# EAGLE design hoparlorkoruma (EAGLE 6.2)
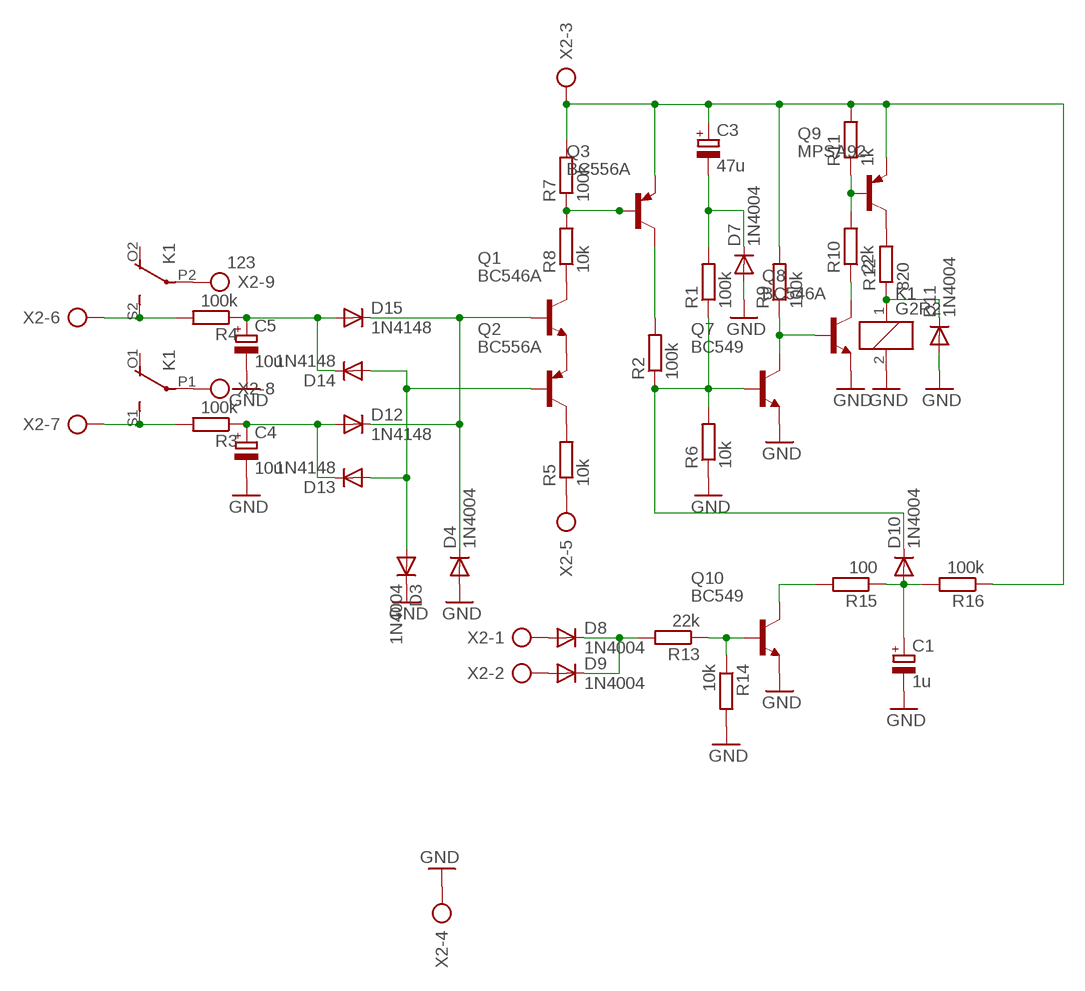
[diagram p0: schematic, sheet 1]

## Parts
C1  1u  CPOL-EUE2.5-6  [E2,5-6]
C3  47u  CPOL-EUE5-8.5  [E5-8,5]
C4  10u  CPOL-EUE2.5-6  [E2,5-6]
C5  10u  CPOL-EUE2.5-6  [E2,5-6]
D3  1N4004  [DO41-10]
D4  1N4004  [DO41-10]
D7  1N4004  [DO41-10]
D8  1N4004  [DO41-10]
D9  1N4004  [DO41-10]
D10  1N4004  [DO41-10]
D11  1N4004  [DO41-10]
D12  1N4148  1N4148DO35-10  [DO35-10]
D13  1N4148  1N4148DO35-7  [DO35-7]
D14  1N4148  1N4148DO35-10  [DO35-10]
D15  1N4148  1N4148DO35-10  [DO35-10]
K1  G2R2  [G2R2]
Q1  BC546A  [TO92-EBC]
Q2  BC556A  [TO92-EBC]
Q3  BC556A  [TO92-EBC]
Q7  BC549  BC546A  [TO92-EBC]
Q8  BC546A  [TO92-EBC]
Q9  MPSA92  MPSA56  [TO92-CBE]
Q10  BC549  BC546A  [TO92-EBC]
R1  100k  R-EU_0207/10  [0207/10]
R2  100k  R-EU_0207/10  [0207/10]
R3  100k  R-EU_0207/10  [0207/10]
R4  100k  R-EU_0207/10  [0207/10]
R5  10k  R-EU_0207/10  [0207/10]
R6  10k  R-EU_0207/10  [0207/10]
R7  100k  R-EU_0207/10  [0207/10]
R8  10k  R-EU_0207/10  [0207/10]
R9  100k  R-EU_0207/10  [0207/10]
R10  22k  R-EU_0207/10  [0207/10]
R11  1k  R-EU_0207/10  [0207/10]
R12  820  R-EU_0411/15  [0411/15]
R13  22k  R-EU_0207/10  [0207/10]
R14  10k  R-EU_0207/10  [0207/10]
R15  100  R-EU_0207/10  [0207/10]
R16  100k  R-EU_0207/10  [0207/10]
X2  123  AK500/9  [AK500/9]

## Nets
GND: C1.- C4.- C5.- D3.C D4.A D7.A D11.A K1.2 Q7.E Q8.E Q10.E R6.1 R14.2 X2.4
N$1: Q1.E Q2.E
N$2: Q2.C R5.2
N$3: Q1.C R8.1
N$4: Q3.B R7.1 R8.2
N$5: C5.+ D14.C D15.A R4.1
N$6: C4.+ D12.A D13.C R3.1
N$7: D4.C D12.C D15.C Q1.B
N$8: D3.A D13.A D14.A Q2.B
N$9: Q7.C Q8.B R9.1
N$10: Q9.B R10.2 R11.1
N$11: C3.+ Q3.E Q9.E R7.2 R9.2 R11.2 R16.1 X2.3
N$12: Q3.C R2.2
N$13: D10.C Q7.B R1.1 R2.1 R6.2
N$14: C3.- D7.C R1.2
N$15: Q9.C R12.2
N$16: Q8.C R10.1
N$17: Q10.B R13.1 R14.1
N$18: D8.C D9.C R13.2
N$19: D8.A X2.1
N$20: Q10.C R15.2
N$21: C1.+ D10.A R15.1 R16.2
N$22: D9.A X2.2
N$23: R5.1 X2.5
N$24: K1.S2(3:S) R4.2 X2.6
N$25: K1.S1(2:S) R3.2 X2.7
N$26: K1.P2(3:P) X2.9
N$27: K1.P1(2:P) X2.8
N$28: D11.C K1.1 R12.1
Unconnected: K1.O1(2:O) K1.O2(3:O)

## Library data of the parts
C1 C3-C5 = rcl:CPOL-EU: POLARIZED CAPACITOR, European symbol
D3 D4 D7-D11 = diode:1N4004: DIODE
D12-D15 = diode:1N4148: DIODE
K1 = relay:G2R2: RELAY 2 x switch, Omron; MF: OMRON COMPONENTS USA; MPN: G2R-2-DC6; OC_FARNELL: unknown; OC_NEWARK: 89C5317
Q1 Q7 Q8 Q10 = transistor-npn:BC546*: NPN Transistor
Q2 Q3 = transistor-pnp:BC556*: PNP Transistror
Q9 = transistor-pnp:MPSA56*: PNP Transistror Source: http://www.fairchildsemi.com/ds/MM/MMBTA56.pdf
R1-R16 = LME49810:R-EU_: RESISTOR, European symbol
X2 = con-ptr500:AK500/9: CONNECTOR; OC_FARNELL: unknown; OC_NEWARK: unknown

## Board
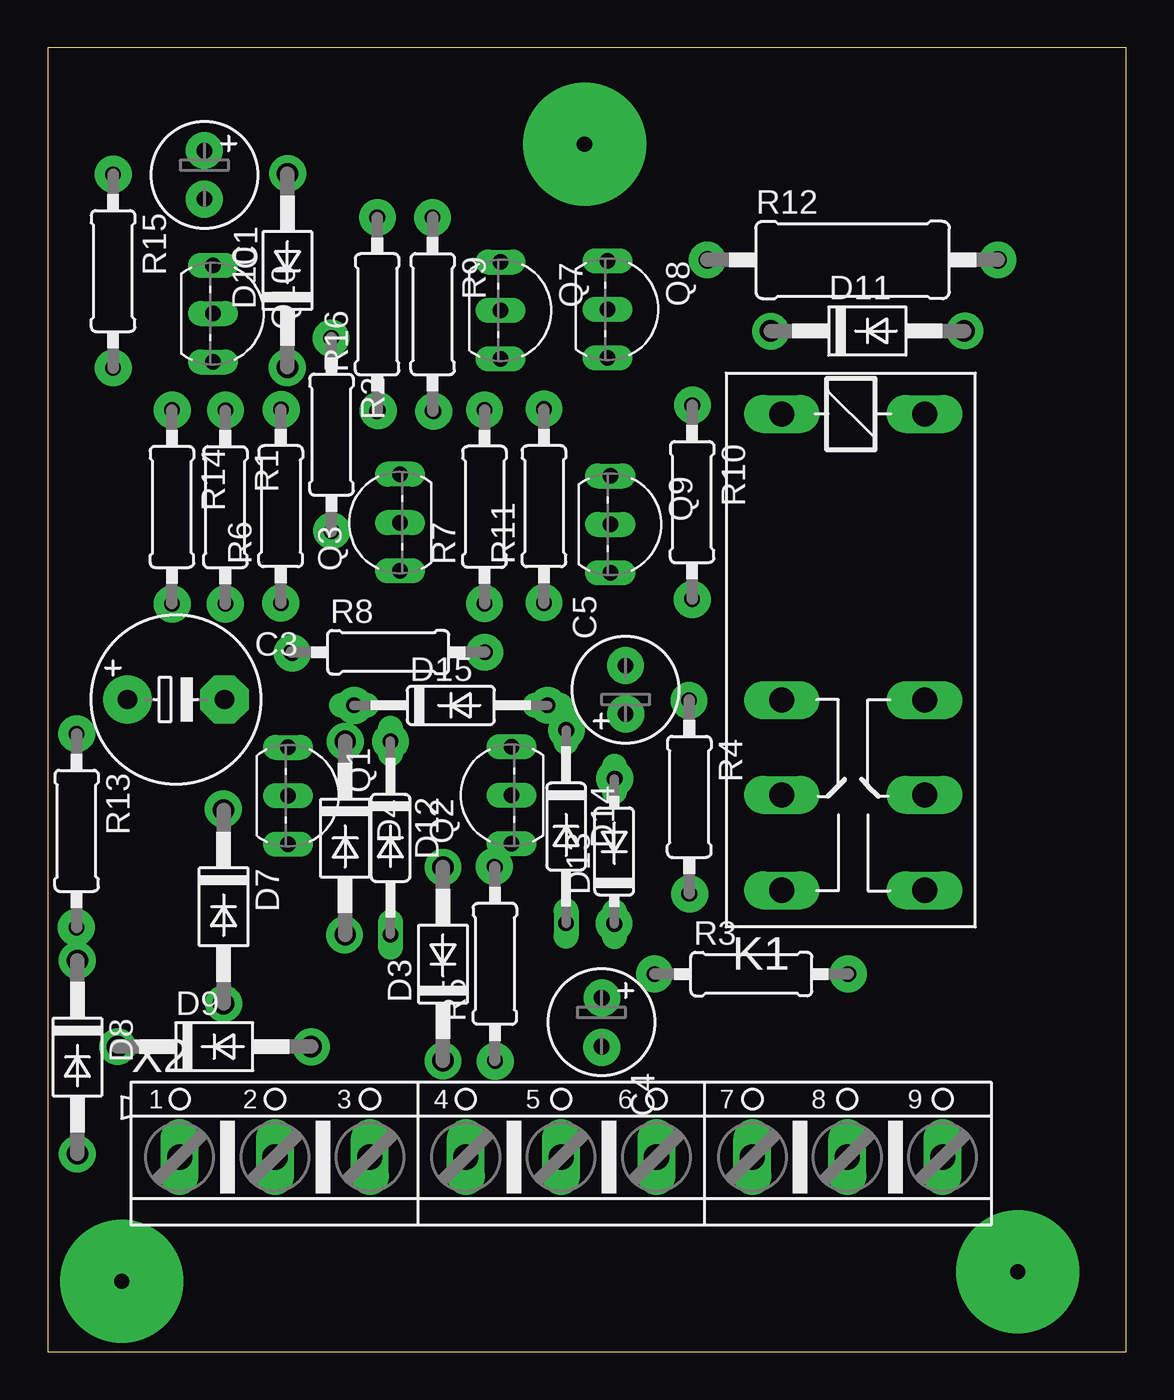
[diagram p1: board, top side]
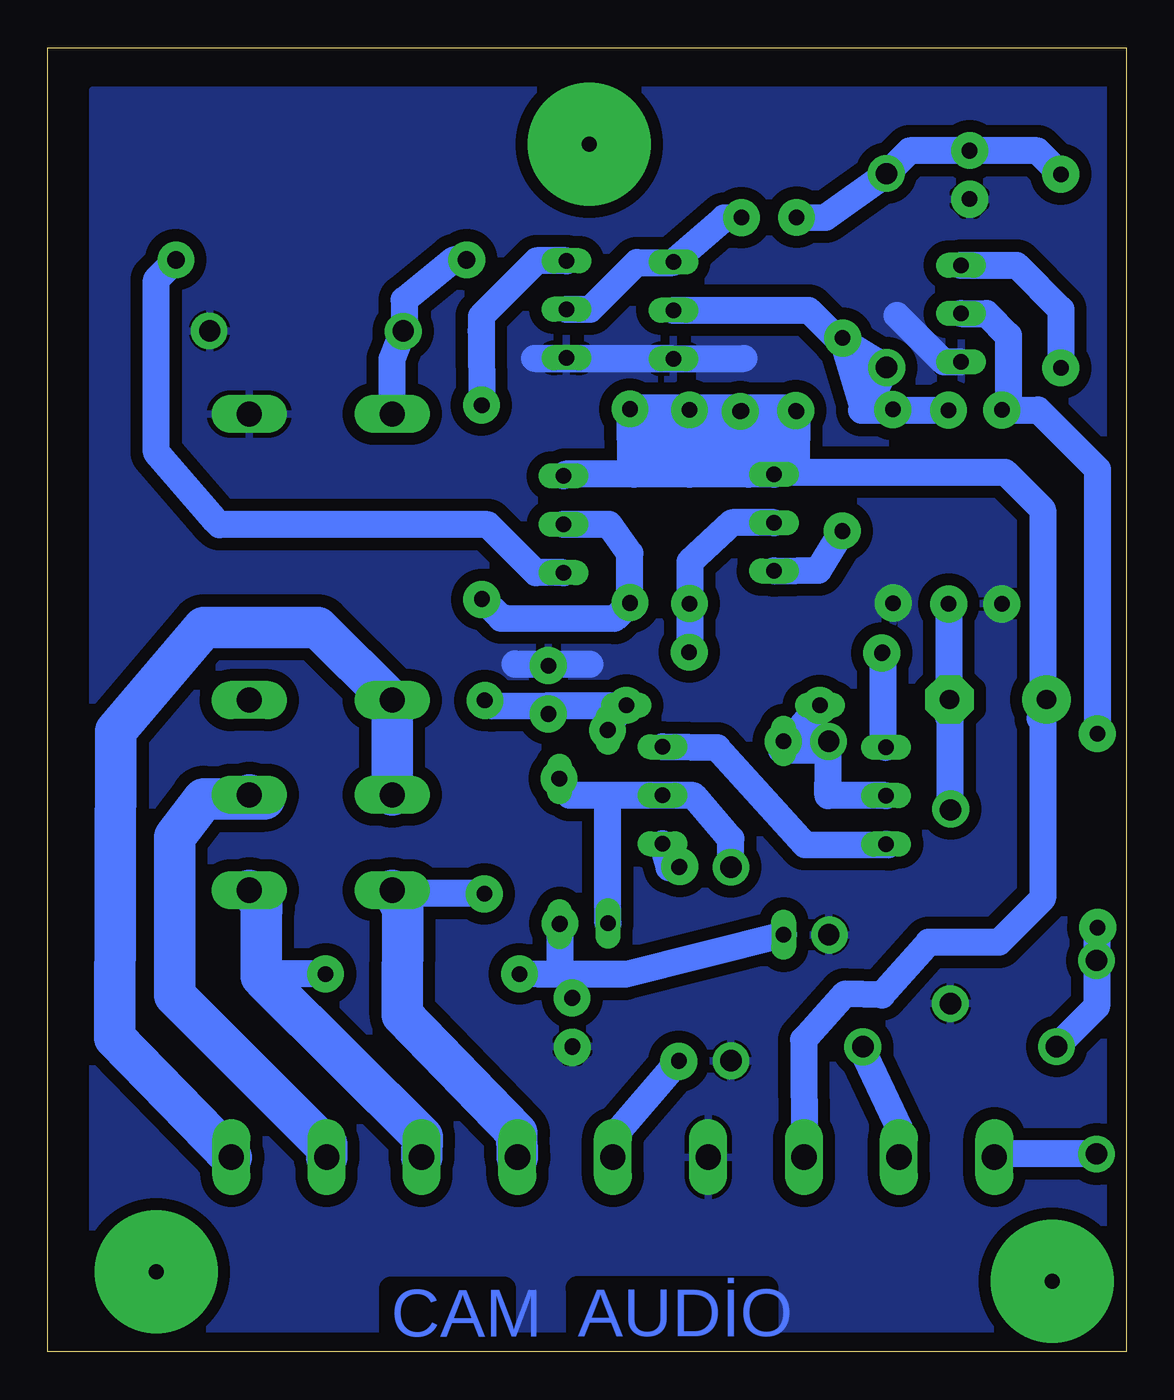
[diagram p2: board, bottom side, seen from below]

Size 56.59 x 68.45 mm. Coordinates in mm from the lower left corner, seen from the top.
Outline: 0,0 56.59,0 56.59,68.45 0,68.45 0,0
Copper layers (1*16): Top 0.035mm / dielectric 1.5mm / Bottom 0.035mm
Design rules: minimum track width 10mil, minimum drill 24mil, track to track 25mil, track to pad 25mil, pad to pad 25mil, via to via 25mil, smd to smd 25mil, copper to edge 40mil, drill to drill 8mil, minimum pad ring 10mil, minimum via ring 8mil, stop-mask expansion 4mil, vias tented up to drill 0mil, thermal gap 10mil

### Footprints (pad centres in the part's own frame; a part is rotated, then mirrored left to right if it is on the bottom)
E2,5-6 = drill 0.813 pad 1.6: + -1.27,0 | drill 0.813 pad 1.6 octagon: - 1.27,0
E5-8,5 = drill 1.016 pad 2.54: + -2.54,0 | drill 1.016 pad 2.54 octagon: - 2.54,0
DO41-10 = drill 1.118: A 5.08,0; C -5.08,0
DO35-10 = drill 0.813 long: A 5.08,0; C -5.08,0
DO35-7 = drill 0.813 long: A 3.81,0; C -3.81,0
G2R2 = drill 1.321 long: 1 -2.54,-3.683; 2 -2.54,3.81; O1 12.471,3.81; O2 12.471,-3.683; P1 17.45,3.81; P2 17.45,-3.683; S1 22.454,3.81; S2 22.454,-3.683
TO92-EBC = drill 0.813 long: B 0,-1.27; C -2.54,-1.27; E 2.54,-1.27
TO92-CBE = drill 0.813 long: B 0,0; C 2.54,0; E -2.54,0
0207/10 = drill 0.813 octagon: 1 -5.08,0; 2 5.08,0
0411/15 = drill 0.914 octagon: 1 -7.62,0; 2 7.62,0
AK500/9 = drill 1.321 long: 1 -20.015,0; 2 -15.011,0; 3 -10.033,0; 4 -5.004,0; 5 0,0; 6 5.004,0; 7 10.033,0; 8 15.011,0; 9 20.015,0

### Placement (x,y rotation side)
C1  8.22,61.77 270 top
C3  6.73,34.24 0 top
C4  29.05,17.31 270 top
C5  30.32,34.75 90 top
D3  20.74,20.36 90 top
D4  15.61,26.97 270 top
D7  9.23,23.36 270 top
D8  1.56,15.47 270 top
D9  8.74,16.02 0 top
D10  12.58,56.75 90 top
D11  43.01,53.58 0 top
D12  17.98,26.98 270 top
D13  29.73,26.26 90 top
D14  27.2,27.57 270 top
D15  21.15,33.93 0 top
K1  42.2,46.68 270 top
Q1  13.88,29.19 270 top
Q2  23.07,29.21 90 top
Q3  17.21,43.52 90 top
Q7  25.03,54.66 270 top
Q8  30.64,54.72 270 top
Q9  29.52,43.43 270 top
Q10  9.94,54.49 270 top
R1  9.32,44.33 270 top
R2  14.89,48.14 270 top
R3  36.92,19.83 0 top
R4  33.66,29.13 270 top
R5  23.46,20.37 90 top
R6  12.23,44.38 90 top
R7  22.92,44.35 90 top
R8  17.86,36.72 0 top
R9  20.2,54.46 270 top
R10  33.81,44.6 270 top
R11  26.04,44.38 90 top
R12  42.23,57.31 0 top
R13  1.52,27.35 270 top
R14  6.52,44.35 270 top
R15  3.43,56.72 270 top
R16  17.29,54.45 90 top
X2  26.94,10.22 0 top

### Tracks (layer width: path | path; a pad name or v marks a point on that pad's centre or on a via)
GND  (via drill 0.8 pad 1.93)
  Bottom 1.422: v6.53,39.25 R14.2 | 12.19,39.26 R6.1 | C4.- v29.07,15.98 | Q7.E 31.04,52.14 20.05,52.14 | 28.13,36.09 32.07,36.09 32.07,36.11 | 8.69,51.95 9.57,51.95 12.03,54.41
  other vias: 12.23,39.3 15.57,21.89 20.74,15.28 30.32,36.02 9.24,18.28 48.13,53.58 8.22,60.49
  pour Bottom: 0.7,66.22 54.23,66.22 54.23,0.51 0.7,0.51
N$1
  Bottom 1.422: Q1.E 12.47,26.61 16.86,26.62 21.45,31.7 Q2.E
N$2
  Bottom 1.422: Q2.C 23.98,25.4 R5.2
N$3
  Bottom 1.422: R8.1 12.78,31.9 arc-90 Q1.C
N$4  (via drill 0.8 pad 1.93)
  Bottom 1.422: Q3.B 20.68,43.52 22.89,41.46 22.89,39.25 | 22.89,39.25 22.89,36.77 R8.2 | R7.1 22.89,39.25
  other vias: 22.92,39.27
N$5
  Bottom 1.422: 27.32,32.77 D14.C 27.2,32.96 D15.A 30.36,33.91 | R4.1 33.28,33.9 30.36,33.91 | C5.+ 30.32,33.87 30.36,33.91
N$6
  Bottom 1.422: D12.A 26.3,19.82 28.37,19.81 | 28.37,19.81 30.82,19.82 31.93,19.84 | 31.93,19.84 R3.1 | D13.C 29.73,19.82 31.93,19.84 | C4.+ 29.05,19.77 28.37,19.81
N$7
  Bottom 1.422: Q1.B 15.66,29.19 D4.C 17.62,32.48 15.77,31.57 | D12.C 15.77,31.57 | D15.C 18.1,31.58 15.77,31.57
N$8
  Bottom 1.422: D3.A 20.74,26.93 22.7,29.2 Q2.B 27.06,29.21 | 27.06,29.21 29.2,29.21 D13.A | D14.A 27.2,29.07 27.06,29.21
N$9
  Bottom 1.422: R9.1 21.1,59.51 Q7.C 23.79,57.17 25.68,57.17 28.13,54.72 Q8.B
N$10
  Bottom 1.422: Q9.B 27.13,43.42 26.04,41.91 R11.1 26.84,38.49 32.55,38.51 32.8,38.51 R10.2
N$11
  Bottom 1.422: 17.39,46.17 18.37,46.17 Q3.E 19.83,46.06 | 17.39,46.17 6.36,46.17 4.39,44.2 4.39,33.12 | 16.89,10.22 X2.3 16.93,16.38 14.77,18.78 12.82,18.73 10.37,21.5 6.69,21.5 4.39,23.8 4.39,33.12 | C3.+ 4.52,33.25 4.39,33.12 | 19.83,46.06 22.91,46.06 | 22.91,46.06 25.82,46.06 | 25.82,46.06 29.43,46.06 Q9.E | R11.2 26.02,46.21 25.82,46.06 | R7.2 22.84,46.13 22.91,46.06 | R9.2 19.91,46.14 19.83,46.06 | R16.1 17.32,46.24 17.39,46.17
N$12
  Bottom 1.422: Q3.C 16.14,41.02 R2.2
N$13  (via drill 0.8 pad 1.93)
  Bottom 1.422: R1.1 12.39,49.41 | 12.39,49.41 13.89,49.41 | 13.89,49.41 13.83,49.63 R2.1 | R6.2 v12.25,49.46 12.34,49.46 12.39,49.41 | 13.89,49.41 13.62,49.68 D10.C 13.07,51.97 | 15.1,53.23 13.07,51.97 | Q7.B 16.66,54.66 13.38,51.38 13.38,51.66 13.07,51.97
N$14
  Bottom 1.422: R1.2 9.32,33.31 C3.- 9.23,34.2 D7.C
N$15
  Bottom 1.422: 47.77,43.58 47.88,43.71 | 47.88,43.71 50.89,47.2 50.89,56.27 R12.2 | 47.88,43.71 47.58,43.41 33.5,43.41 30.98,40.89 Q9.C
N$16
  Bottom 1.422: R10.1 33.85,53.58 33.84,53.59 33.84,54.35 30.93,57.26 Q8.C
N$17
  Bottom 1.422: 6.39,49.56 R14.1 | R14.1 4.62,49.43 1.52,46.33 R13.1 | Q10.B 7.33,54.49 6.18,53.34 6.18,49.77 R14.1
N$18
  Bottom 1.422: D9.C 1.56,18.12 D8.C 1.56,22.23 R13.2
N$19
  Bottom 1.422: D8.A 6.75,10.39 X2.1
N$20
  Bottom 1.422: Q10.C 5.76,57.03 3.43,54.7 R15.2
N$21
  Bottom 1.422: 12.85,61.75 D10.A | R16.2 15.78,59.54 D10.A | R15.1 4.67,63.04 C1.+ 11.37,63.04 D10.A
N$22
  Bottom 1.422: 11.93,10.34 X2.2 11.89,10.26 11.89,11.7 13.66,15.47 D9.A
N$23
  Bottom 1.422: R5.1 26.94,11.23 X2.5
N$24
  Bottom 1.422: R4.2 37.93,24.05 38.23,23.74
  Bottom 2.184: X2.6 31.97,11.49 37.98,17.68 37.95,23.26 38.23,23.74 K1.S2
N$25
  Bottom 1.422: 45.37,23.13 45.39,23.11 | R3.2 44.69,19.83 45.12,19.41
  Bottom 2.184: X2.7 36.94,11.29 45.12,19.41 45.39,19.7 45.39,23.11 | K1.S1 45.37,23.59 45.37,23.13
N$26
  Bottom 2.184: K1.P2 38.52,34.13 42.41,38.02 48.41,38.02 53.03,32.58 53.06,16.48 X2.9
N$27
  Bottom 2.184: X2.8 41.95,10.74 | 41.95,10.74 41.95,10.88 | K1.P1 45.22,29.02 48.41,29.02 49.91,27.02 49.91,18.7 41.95,10.74
N$28  (via drill 0.8 pad 1.93)
  Bottom 1.422: K1.1 38.52,52.1 D11.C 37.89,53.62 37.89,55.2 35.28,57.31 R12.1
  other vias: 34.61,57.31
N$29  (via drill 0.8 pad 6.45)
  other vias: 3.89,3.7
N$30  (via drill 0.8 pad 6.45)
  other vias: 50.89,4.2
N$31  (via drill 0.8 pad 6.45)
  other vias: 28.17,63.38
N$32  (via drill 0.8 pad 1.93)
  other vias: 1.5,22.27
N$33  (via drill 0.8 pad 1.93)
  other vias: 1.52,32.44
N$34  (via drill 0.8 pad 1.93)
  other vias: 6.54,49.43
N$35  (via drill 0.8 pad 1.93)
  other vias: 9.33,49.43
N$36  (via drill 0.8 pad 1.93)
  other vias: 14.87,53.21
N$37  (via drill 0.8 pad 1.93)
  other vias: 17.34,49.4
N$38  (via drill 0.8 pad 1.93)
  other vias: 20.26,49.36
N$39  (via drill 0.8 pad 1.93)
  other vias: 12.57,51.66
N$40  (via drill 0.8 pad 1.93)
  other vias: 3.44,51.64
N$41  (via drill 0.8 pad 1.93)
  other vias: 3.44,61.81
N$42  (via drill 0.8 pad 1.93)
  other vias: 12.6,61.85
N$43  (via drill 0.8 pad 1.93)
  other vias: 17.3,59.54
N$44  (via drill 0.8 pad 1.93)
  other vias: 20.19,59.53
N$45  (via drill 0.8 pad 1.93)
  other vias: 33.83,49.69
N$46  (via drill 0.8 pad 1.93)
  other vias: 26.04,49.49
N$47  (via drill 0.8 pad 1.93)
  other vias: 42.01,19.84
N$48  (via drill 0.8 pad 1.93)
  other vias: 22.92,49.44
N$49  (via drill 0.8 pad 1.93)
  other vias: 22.93,36.72
N$50  (via drill 0.8 pad 1.93)
  other vias: 26.04,39.32
N$51  (via drill 0.8 pad 1.93)
  other vias: 14.9,43.09
N$52  (via drill 0.8 pad 1.93)
  other vias: 9.32,39.25
N$53  (via drill 0.8 pad 1.93)
  other vias: 1.56,20.55
N$54  (via drill 0.8 pad 1.93)
  other vias: 13.83,16
N$55  (via drill 0.8 pad 1.93)
  other vias: 1.56,10.38
N$56  (via drill 0.8 pad 1.93)
  other vias: 3.66,16.02
N$57  (via drill 0.8 pad 1.93)
  other vias: 23.48,15.25
N$58  (via drill 0.8 pad 1.93)
  other vias: 33.82,39.49
N$59  (via drill 0.8 pad 1.93)
  other vias: 20.74,25.44
N$60  (via drill 0.8 pad 1.93)
  other vias: 23.43,25.48
N$61  (via drill 0.8 pad 1.93)
  other vias: 49.86,57.31
N$62  (via drill 0.8 pad 1.93)
  other vias: 29.76,30.09
N$63  (via drill 0.8 pad 1.93)
  other vias: 29.71,22.48
N$64  (via drill 0.8 pad 1.93)
  other vias: 31.84,19.83
N$65  (via drill 0.8 pad 1.93)
  other vias: 15.62,32.04
N$66  (via drill 0.8 pad 1.93)
  other vias: 17.99,32.03
N$67  (via drill 0.8 pad 1.93)
  other vias: 16.08,33.93
N$68  (via drill 0.8 pad 1.93)
  other vias: 26.24,33.94
N$69  (via drill 0.8 pad 1.93)
  other vias: 30.33,33.47
N$70  (via drill 0.8 pad 1.93)
  other vias: 27.22,32.63
N$71  (via drill 0.8 pad 1.93)
  other vias: 33.65,34.18
N$72  (via drill 0.8 pad 1.93)
  other vias: 12.83,36.67
N$73  (via drill 0.8 pad 1.93)
  other vias: 9.21,28.49
N$74  (via drill 0.8 pad 1.93)
  other vias: 29.08,18.57
N$75
  Bottom 1.422: 17.33,49.53 17.34,49.54 25.85,49.54 25.67,48.42 17.33,48.42 17.33,47.39 25.59,47.39 25.59,47.43 25.63,47.43 25.63,47.5 25.49,47.5
N$76  (via drill 0.8 pad 1.93)
  other vias: 8.22,63.05
N$77  (via drill 0.8 pad 1.93)
  other vias: 37.93,53.56
N$78  (via drill 0.8 pad 1.93)
  other vias: 33.68,24.03

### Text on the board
Bottom: AUDİO | CAM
